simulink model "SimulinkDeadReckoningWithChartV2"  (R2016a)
settings: Solver=FixedStepAuto  StartTime=0.0  StopTime=inf  RelTol=1e-3
libraries: miniQ x2

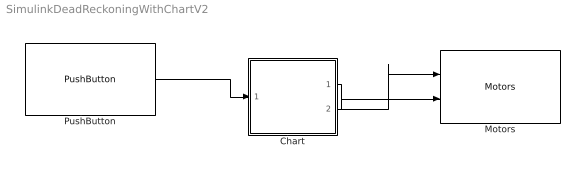
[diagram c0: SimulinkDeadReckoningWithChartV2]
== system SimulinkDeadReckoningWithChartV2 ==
  Chart : Stateflow chart  TreatAsAtomicUnit=on
  Motors : miniQ/Motors  flipLeft=off  flipRight=off
  PushButton : miniQ/PushButton  sampleTime_dd=0.1  debug_dd=off
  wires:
  Chart/2(l) -> Motors/1
  Chart/1(r) -> Motors/2
  PushButton/1 -> Chart/1(button)

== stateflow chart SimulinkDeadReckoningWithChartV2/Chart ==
  state Experiment with changing the "after(int,sec) function and also the values for r and l to get the dead reckoing patter you desire [group]
  state InitialState
    entry: r=0
    l=0
  state Stop
    entry: r=0
    l=0
  state Forward3
    entry: r=255
    l=255
  state Left3
    entry: r=255
    l=-255
  state Forward
    entry: r=255
    l=255
  state Forward2
    entry: r=255
    l=255
  state Left
    entry: r=255
    l=-255
  state Forward1
    entry: r=255
    l=255
  state Left2
    entry: r=255
    l=-255
  (default) -> InitialState
  Stop -> InitialState
  Left3 -> Forward3 : after(.2,sec)
  Forward3 -> Stop : after(.2,sec)
  InitialState -> Forward : [button==1]
  Forward2 -> Left3 : after(0.5,sec)
  Forward -> Left : after(0.7,sec)
  Left2 -> Forward2 : after(.2,sec)
  Left -> Forward1 : after(.2,sec)
  Forward1 -> Left2 : after(.5,sec)
  data: r output; l output; button input
